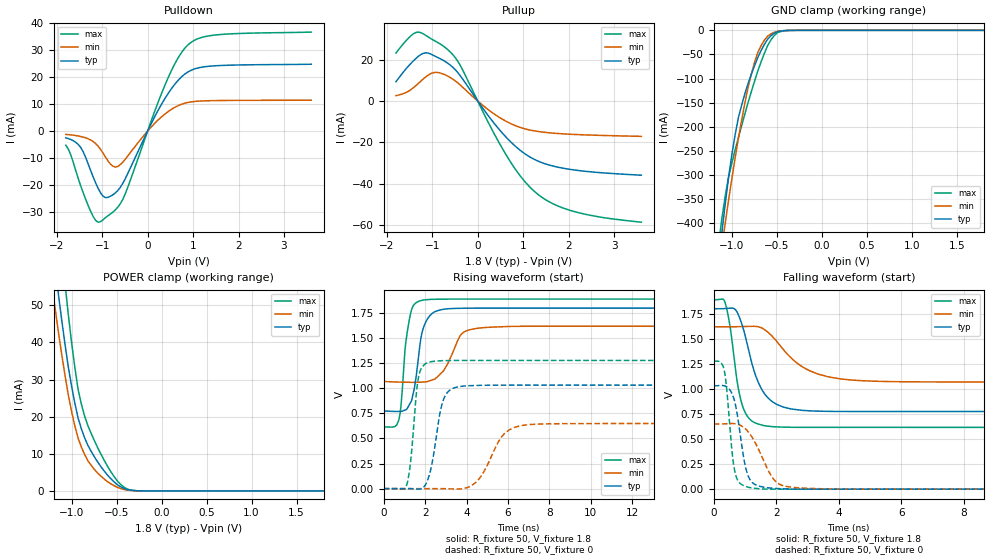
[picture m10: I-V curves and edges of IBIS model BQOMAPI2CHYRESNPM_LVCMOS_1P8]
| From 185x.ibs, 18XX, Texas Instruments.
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|   Model Cell BQOMAPI2CHYRESNPM_LVCMOS_1P8
|BQOMAPI2CHYRESNPM_LVCMOS_1P8
[Model]   BQOMAPI2CHYRESNPM_LVCMOS_1P8
Model_type   I/O
Polarity   Non-Inverting
Enable   Active-Low
Vinl =  0.54
Vinh =  1.26
Cref =  15.0000PF
Rref =  150.0000
Vref =  0V
Vmeas =  0.9
C_comp   3.856143p   3.721565p   3.857354p
[Model Spec]
Vinl   0.54   0.486   0.567
Vinh   1.26   1.134   1.323
[Temperature Range]   25   125   -40
[Voltage Range]   1.8   1.62   1.89
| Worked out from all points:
|   slope of the pulldown table from 0 to 0.27 V, typ, clamps not added: 30.5 ohm
|   slope of the pullup table from 0 to 0.27 V, typ, clamps not added: 32.9 ohm
|   GND clamp passes 1 mA (typ) near -0.43 V on its own axis
|   POWER clamp passes 1 mA (typ) near -0.44 V on its own axis
|   rising waveform, R_fixture 50, V_fixture 1.8: 20-80 % time 441ps typ, 753ps min, 340ps max; typ from 0.774 V to 1.8 V
|   rising waveform, R_fixture 50, V_fixture 0: 20-80 % time 506ps typ, 990ps min, 322ps max; typ from 0 V to 1.03 V
|   falling waveform, R_fixture 50, V_fixture 1.8: 20-80 % time 615ps typ, 1.17ns min, 366ps max; typ from 1.8 V to 0.775 V
|   falling waveform, R_fixture 50, V_fixture 0: 20-80 % time 322ps typ, 623ps min, 223ps max; typ from 1.03 V to 0 V
| Nom Voltages:
|   BIASFET=1.8, VDDS=1.8, VDDU=1.2, BUS_VDD=0, VSS=0, VSSS=0
| Min Voltages:
|   BIASFET=1.62, VDDS=1.62, VDDU=1.08, BUS_VDD=0, VSS=0, VSSS=0
| Max Voltages:
|   BIASFET=1.89, VDDS=1.89, VDDU=1.32, BUS_VDD=0, VSS=0, VSSS=0
[POWER_clamp]
|   voltage   I(typ)   I(min)   I(max)
-1.8V     219.8mA    174.8mA    280.3mA
-1.218V   68.59mA    55.65mA    92.28mA
-1.182V   60.61mA    49.1mA     82.82mA
-1.145V   52.95mA    42.72mA    73.55mA
-1.073V   39.56mA    31.2mA     56.02mA
-1.036V   33.49mA    25.92mA    47.65mA
-963.6mV  23.72mA    17.61mA    33.37mA
-890.9mV  16.76mA    11.84mA    23.42mA
-781.8mV  10.67mA    6.886mA    15.5mA
-563.6mV  3.296mA    1.922mA    5.2mA
-309.1mV  100.1uA    71.54uA    112.3uA
1.8V      -2.406uA   -6.294uA   -2.119uA
[Pulldown]
|   voltage   I(typ)   I(min)   I(max)
-1.8V     -2.485mA   -1.225mA   -5.216mA
-1.473V   -6.029mA   -1.985mA   -20.2mA
-1.2V     -16.85mA   -3.814mA   -31.52mA
-1.036V   -22.81mA   -6.704mA   -33.52mA
-872.7mV  -24.5mA    -11mA      -31.32mA
-654.5mV  -21.95mA   -13.04mA   -28.11mA
-490.9mV  -17.58mA   -10.38mA   -23.15mA
381.8mV   12.07mA    6.333mA    17.03mA
654.5mV   18.46mA    9.287mA    26.62mA
872.7mV   21.73mA    10.55mA    31.65mA
1.473V    24.15mA    11.29mA    35.52mA
3.6V      24.74mA    11.45mA    36.63mA
[Pullup]
|   voltage   I(typ)   I(min)   I(max)
-1.8V     9.335mA    2.582mA    23.2mA
-1.473V   18.13mA    5.455mA    31.51mA
-1.309V   21.56mA    8.475mA    33.33mA
-981.8mV  22.15mA    13.68mA    29.53mA
-600mV    17.28mA    11.3mA     23.62mA
-381.8mV  12.17mA    7.689mA    17.11mA
272.7mV   -8.276mA   -4.854mA   -12.07mA
709.1mV   -19.38mA   -10.74mA   -29.03mA
1.091V    -26.28mA   -13.72mA   -40.31mA
1.418V    -29.84mA   -14.98mA   -46.64mA
2.236V    -33.64mA   -16.26mA   -54.08mA
3.6V      -35.85mA   -17.07mA   -58.57mA
[GND_clamp]
|   voltage   I(typ)   I(min)   I(max)
-1.8V     -1.732A    -1.456A    -1.797A
-1.145V   -477.7mA   -496.1mA   -441.1mA
-1.109V   -417.6mA   -447.5mA   -389.2mA
-1.073V   -360.2mA   -399.8mA   -343.9mA
-1V       -259mA     -308.9mA   -276.1mA
-927.3mV  -181.9mA   -224.8mA   -222.9mA
-818.2mV  -110mA     -117.7mA   -149.4mA
-709.1mV  -55.63mA   -44.94mA   -83.51mA
-563.6mV  -11.08mA   -7.285mA   -19.53mA
-490.9mV  -2.699mA   -1.926mA   -4.617mA
-381.8mV  -277uA     -254.4uA   -403uA
1.8V      5.734uA    8.877uA    5.605uA
[Ramp]
| variable   typ   min   max
dV/dt_f 0.61905018/0.61756056n  0.3338547/1.1749987n 0.76833854/0.36786265n
dV/dt_r 0.62207612/0.50899872n 0.39191715/0.9956608n 0.77011338/0.3239941n
R_load = 50.0000
[Rising Waveform]
R_fixture = 50
V_fixture = 1.8
V_fixture_min = 1.62
V_fixture_max = 1.89
|   time   V(typ)   V(min)   V(max)
0s        774.2mV    1.069V     616.6mV
730.7ps   769.7mV    1.062V     682.9mV
835.3ps   770.6mV    1.062V     821mV
1.058ns   785.7mV    1.061V     1.438V
1.351ns   878.7mV    1.06V      1.785V
1.847ns   1.552V     1.062V     1.878V
2.49ns    1.766V     1.095V     1.888V
3.738ns   1.798V     1.537V     1.89V
4.672ns   1.8V       1.602V     1.89V
25.02ns   1.8V       1.62V      1.89V
[Rising Waveform]
R_fixture = 50
V_fixture = 0
V_fixture_min = 0
V_fixture_max = 0
|   time   V(typ)   V(min)   V(max)
0s        0V         0V         0V
1.094ns   0V         0V         26.7mV
1.303ns   0V         0V         271.5mV
1.676ns   -4.803mV   0V         1.104V
2.211ns   141.1mV    0V         1.262V
2.86ns    872.3mV    0V         1.276V
3.609ns   1.016V     -3.48mV    1.278V
4.44ns    1.028V     60.93mV    1.278V
6.665ns   1.032V     629.7mV    1.278V
25.14ns   1.032V     649.7mV    1.278V
[Falling Waveform]
R_fixture = 50
V_fixture = 1.8
V_fixture_min = 1.62
V_fixture_max = 1.89
|   time   V(typ)   V(min)   V(max)
0s        1.8V       1.62V      1.89V
391.1ps   1.803V     1.62V      1.831V
528.7ps   1.806V     1.62V      1.61V
699.5ps   1.789V     1.621V     1.181V
942.6ps   1.604V     1.623V     809.9mV
1.301ns   1.169V     1.625V     665mV
1.675ns   932.1mV    1.581V     630.8mV
2.922ns   784.7mV    1.205V     616.8mV
4.585ns   775mV      1.085V     616.6mV
25.02ns   775.1mV    1.069V     616.6mV
[Falling Waveform]
R_fixture = 50
V_fixture = 0
V_fixture_min = 0
V_fixture_max = 0
|   time   V(typ)   V(min)   V(max)
0s        1.032V     649.7mV    1.278V
344.5ps   1.031V     652.3mV    1.171V
414.5ps   1.021V     653.7mV    999.4mV
596.2ps   945.3mV    655.4mV    336.6mV
713.7ps   812.7mV    651.8mV    127.8mV
1.002ns   241.3mV    605.4mV    29.37mV
1.209ns   73.74mV    526.8mV    12.55mV
1.926ns   8.24mV     95.65mV    0V
2.752ns   0V         12.38mV    0V
25.14ns   0V         0V         0V
